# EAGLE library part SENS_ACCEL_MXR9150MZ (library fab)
3-axis 3.3V accelerometer
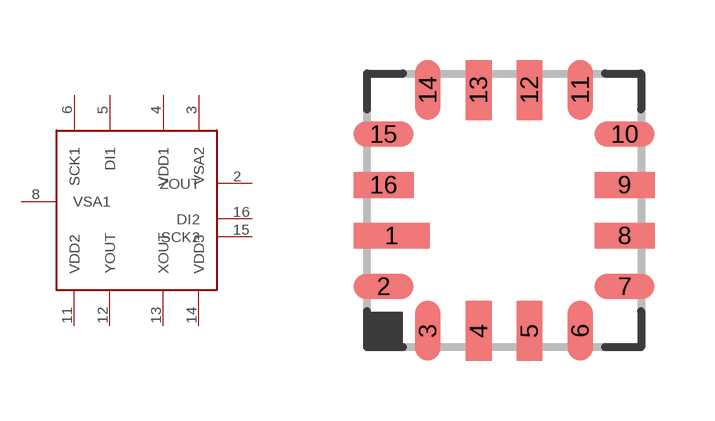
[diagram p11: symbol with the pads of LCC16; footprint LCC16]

Designator prefix -

## SENS_ACCEL_MXR9150MZ  [LCC16]
2  ZOUT
3  VSA2
4  VDD1
5  DI1
6  SCK1
8  VSA1
11  VDD2
12  YOUT
13  XOUT
14  VDD3
15  SCK2
16  DI2

## Footprint LCC16 (pad centres in mm)
LCC16 Package Source: http://www.memsic.com/data/products/MXR9500G&M/MXR9500G&M.pdf
smd 1.9 x 0.64: 1 -2.815,-0.635
smd 1.5 x 0.64: 2 -3.015,-1.905; 7 3.015,-1.905; 8 3.015,-0.635; 9 3.015,0.635; 10 3.015,1.905; 15 -3.015,1.905; 16 -3.015,0.635
smd 0.64 x 1.5: 3 -1.905,-3.015; 4 -0.635,-3.015; 5 0.635,-3.015; 6 1.905,-3.015; 11 1.905,3.015; 12 0.635,3.015; 13 -0.635,3.015; 14 -1.905,3.015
